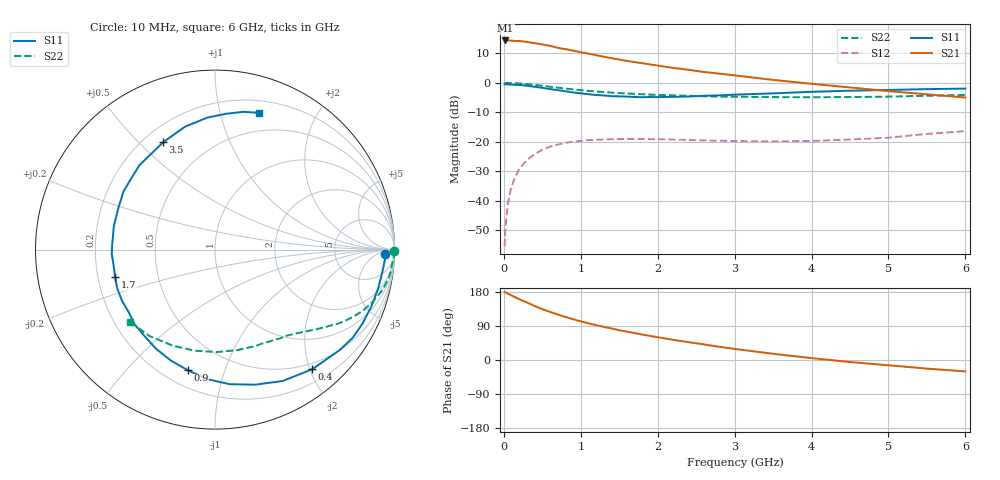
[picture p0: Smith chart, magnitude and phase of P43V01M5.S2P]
! SIEMENS Small Signal Semiconductors
! BFP182
! Si NPN RF Bipolar Junction Transistor in SOT143
! VCE = 3 V  IC = 1.5 mA
! Common Emitter S-Parameters:  March  1996
# GHz  S  MA  R  50
!  f  S11  S21  S12  S22
! GHz  MAG  ANG  MAG  ANG  MAG  ANG  MAG  ANG
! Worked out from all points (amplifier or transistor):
!   36 points, 10 MHz to 6 GHz, reference 50 ohm
!   highest |S21| = 14.4 dB at 20 MHz (marker M1)
!   |S21| within 3 dB of that: start of sweep to 810.2 MHz
!   unconditionally stable (mu >= 1): 2.386 GHz to end of sweep
!   at 250 MHz: K = 0.11, MSG = 20.9 dB, |S12| = -27.7 dB
!   at 1.4 GHz: K = 0.61, MSG = 13.7 dB, |S12| = -19.1 dB
!   at 6 GHz: K = 1.02, MAG = 4.8 dB, |S12| = -16.4 dB
!   S11 on the Smith chart (normalised r, x): 10 MHz: 30, -13; 400 MHz: 0.40, -2.04; 900 MHz: 0.30, -0.75; 1.7 GHz: 0.27, -0.12; 3.5 GHz: 0.28, +0.59; 6 GHz: 0.31, +1.32
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0.01  0.9459 -1.4  5.236 179.4  0.0017 81.8  0.998 -0.5
0.02  0.9495 -2.8  5.243 178.7  0.0034 88.4  0.9955 -1.0
0.05  0.9423 -6.6  5.235 175.2  0.0087 88.8  0.9964 -2.5
0.1  0.935 -13.1  5.202 170.4  0.0174 81.0  0.9892 -5.0
0.15  0.9268 -20.1  5.135 165.5  0.0259 77.9  0.9864 -7.5
0.2  0.9196 -26.4  5.139 160.5  0.0342 74.8  0.9773 -9.9
0.25  0.9116 -32.5  5.044 155.9  0.0414 70.6  0.9659 -12.3
0.4  0.859 -50.9  4.73 142.5  0.0619 60.2  0.9242 -18.5
0.5  0.8236 -62.7  4.486 134.2  0.0735 53.7  0.8928 -22.3
0.6  0.7853 -73.4  4.257 127.0  0.0828 48.0  0.8603 -25.5
0.7  0.7543 -83.8  3.942 120.2  0.0896 42.9  0.8303 -28.3
0.9  0.6884 -102.8  3.521 107.7  0.1006 34.4  0.7765 -32.8
1.1  0.6429 -120.8  3.134 96.7  0.107 27.7  0.7326 -36.7
1.4  0.5941 -143.9  2.623 83.1  0.1107 19.5  0.6849 -41.6
1.7  0.5772 -164.7  2.252 71.1  0.1121 14.3  0.6499 -45.9
1.9  0.5757 -177.5  2.058 63.7  0.111 11.6  0.6324 -48.8
2.2  0.5788 166.6  1.794 53.3  0.1095 8.8  0.6149 -53.3
2.8  0.6137 138.9  1.435 34.9  0.1045 6.7  0.5855 -63.4
3.5  0.6641 115.8  1.123 16.4  0.1018 7.8  0.5736 -77.4
4.5  0.7366 93.3  0.837 -5.4  0.1096 13.6  0.5747 -101.4
5.5  0.7833 78.5  0.64 -22.7  0.1365 17.2  0.6045 -127.2
6  0.8004 72.2  0.565 -30.2  0.1517 14.8  0.6226 -139.9
